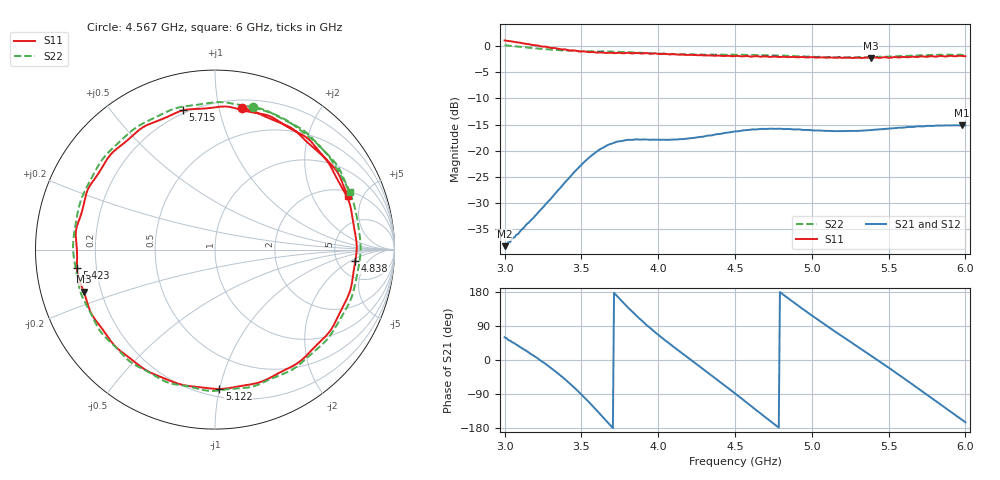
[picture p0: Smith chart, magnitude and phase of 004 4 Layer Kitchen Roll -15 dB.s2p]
!  04/11/2025  14:13:18
! Ref Plane: 0.000 mm
# MHZ S MA R  50
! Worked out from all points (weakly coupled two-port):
!   401 points, 3 GHz to 6 GHz, reference 50 ohm
!   highest |S21| = -15.12 dB at 5.978 GHz (marker M1); lowest = -38.2 dB at 3 GHz (marker M2)
!   lowest |S11| = -2.3 dB at 5.385 GHz (marker M3), VSWR 7.61, Z = 6.73 - j7.66 ohm
!   |S11| at or under -10 dB: nowhere
!   |S22| runs from -2.2 to 0.2 dB; largest |S21 - S12| = 0.0044
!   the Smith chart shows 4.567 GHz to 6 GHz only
!   S11 on the Smith chart (normalised r, x): 4.567 GHz: 0.27, +1.18; 4.838 GHz: 7.49, -2.40; 5.122 GHz: 0.25, -1.00; 5.423 GHz: 0.13, -0.06; 5.715 GHz: 0.18, +0.78; 6 GHz: 2.31, +3.82
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3000  1.129 -115.2  0.01232 59.9  0.01237 61.2  1.018 -117.5
3270  0.983 177.0  0.03134 -11.4  0.03112 -9.8  0.9335 174.6
3390  0.9295 139.4  0.04948 -49.6  0.04959 -48.8  0.9099 135.9
3502.5  0.8886 96.8  0.07422 -92.1  0.07424 -91.3  0.893 93.2
3600  0.8644 55.3  0.09843 -133.1  0.09873 -132.5  0.8868 52.6
3735  0.8605 -5.6  0.1226 167.3  0.1229 168.6  0.8794 -5.8
3862.5  0.8584 -58.0  0.1284 115.1  0.1291 116.6  0.8651 -56.6
4005  0.8383 -107.8  0.1272 65.2  0.127 66.3  0.8446 -106.2
4237.5  0.8179 -179.5  0.1332 -7.2  0.1332 -5.9  0.829 -179.4
4357.5  0.8078 144.5  0.1414 -43.7  0.1418 -42.3  0.8278 143.0
4500  0.8024 100.1  0.1531 -88.4  0.1539 -87.4  0.8231 96.9
4567.5  0.8014 79.0  0.1573 -109.8  0.1574 -108.9  0.8201 74.9
4710  0.7926 35.0  0.1619 -154.8  0.1622 -153.9  0.8139 29.2
4837.5  0.7842 -4.5  0.1617 165.4  0.1616 166.6  0.8035 -10.4
5002.5  0.7822 -53.9  0.1567 116.9  0.1568 117.8  0.7938 -58.9
5122.5  0.7768 -88.2  0.1548 83.2  0.1549 84.1  0.7877 -92.7
5385  0.7676 -162.3  0.1578 11.7  0.1583 12.7  0.7853 -164.2
5422.5  0.776 -172.4  0.1595 1.3  0.1597 2.3  0.7853 -174.9
5505  0.771 163.7  0.1631 -21.5  0.1638 -20.4  0.7947 162.3
5715  0.7964 102.9  0.1707 -81.7  0.1711 -80.4  0.8173 103.6
5977.5  0.8034 29.0  0.1753 -157.5  0.1762 -156.3  0.8213 30.1
6000  0.7989 22.0  0.1747 -164.4  0.1752 -163.3  0.817 23.0
